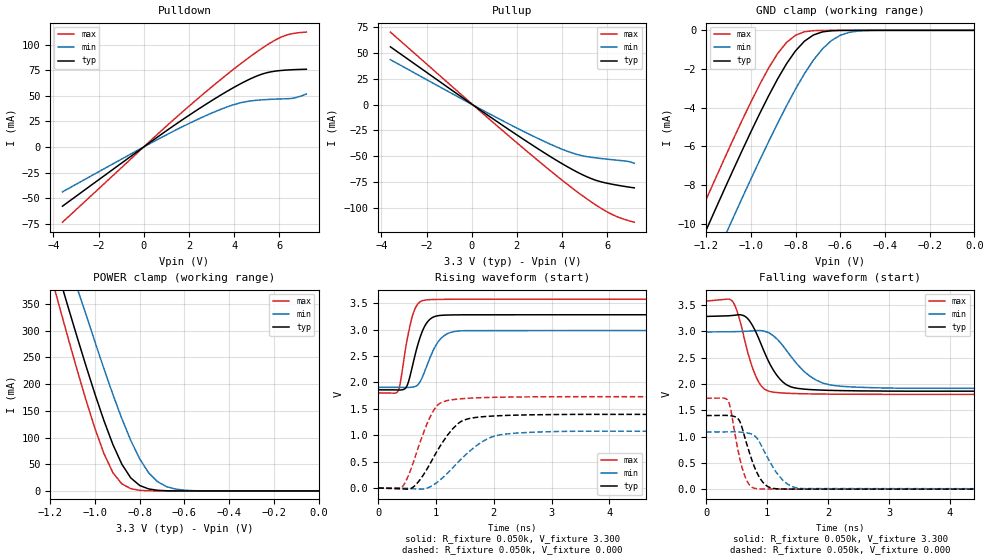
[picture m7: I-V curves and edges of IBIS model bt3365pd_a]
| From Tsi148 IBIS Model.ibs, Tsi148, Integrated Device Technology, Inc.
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|   MODEL bt3365pd_a
[Model]   bt3365pd_a
Model_type   I/O
Vinl  = 0.8V
Vinh  = 2.0V
Vref  = 0.0V
Rref  = 1k
Cref  = 10pF
Vmeas = 1.65V
| Values for delay from A to PAD (Tdo) are determined using
| Vref, Cref, Rref, and Vmeas.
|   INPUT TRANSITION ON DRIVER INPUT = 0.1ns
|   typ   min   max
| Tdo (rise)   1.63n   1.15n   2.34n
| Tdo (fall)   1.53n   1.15n   2.10n
|   INPUT TRANSITION ON DRIVER INPUT = 1.0ns
|   typ   min   max
| Tdo (rise)   1.84n   1.30n   2.60n
| Tdo (fall)   1.63n   1.25n   2.21n
|   typ   min   max
C_comp   1.29pF   1.27pF  1.30pF
[Temperature Range]   50.00   125.00   0.00
[Voltage Range]   3.300   3.000   3.600
|   typ   min   max
|[Supply]   VDD   1.80   1.65   1.95
|[Supply]   VDD330   3.30   3.00   3.60
[Add Submodel]
| Submodel Name   Mode
Up.bt3365pd_a   Non-Driving
Dn.bt3365pd_a   Non-Driving
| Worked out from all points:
|   slope of the pulldown table from 0 to 0.495 V, typ, clamps not added: 62.8 ohm
|   slope of the pullup table from 0 to 0.495 V, typ, clamps not added: 65.6 ohm
|   GND clamp passes 1 mA (typ) near -0.80 V on its own axis
|   POWER clamp passes 1 mA (typ) near -0.71 V on its own axis
|   rising waveform, R_fixture 0.050k, V_fixture 3.300: 20-80 % time 220ps typ, 268ps min, 176ps max; typ from 1.86 V to 3.29 V
|   falling waveform, R_fixture 0.050k, V_fixture 3.300: 20-80 % time 364ps typ, 510ps min, 262ps max; typ from 3.29 V to 1.86 V
|   rising waveform, R_fixture 0.050k, V_fixture 0.000: 20-80 % time 488ps typ, 655ps min, 355ps max; typ from 0 V to 1.4 V
|   falling waveform, R_fixture 0.050k, V_fixture 0.000: 20-80 % time 246ps typ, 336ps min, 182ps max; typ from 1.4 V to 0 V
[Pullup]   | Note: Vtable = Vcc - Vout
| Voltage   I(typ)   I(min)   I(max)
-3.6V     56.12mA    43.64mA    70.43mA
1.37V     -20.18mA   -15.67mA   -25.27mA
3.02V     -44.1mA    -33.79mA   -55.87mA
4.12V     -58.9mA    -44.36mA   -75.46mA
4.67V     -65.54mA   -48.47mA   -84.72mA
5.11V     -70.21mA   -50.58mA   -91.74mA
5.88V     -75.84mA   -52.74mA   -102.7mA
6.54V     -78.66mA   -54.24mA   -109.8mA
6.87V     -79.84mA   -55mA      -112.2mA
7.2V      -80.88mA   -56.98mA   -114.3mA
[Pulldown]   | Note: Vtable = Vout
| Voltage   I(typ)   I(min)   I(max)
-3.6V     -57.91mA   -43.93mA   -73.58mA
1.35V     21.13mA    15.75mA    27.16mA
2.89V     43.61mA    31.96mA    56.47mA
3.99V     58.18mA    41.33mA    76.18mA
4.54V     64.64mA    44.3mA     85.49mA
5.09V     70.03mA    45.79mA    94.25mA
5.53V     72.96mA    46.44mA    100.7mA
5.97V     74.5mA     46.85mA    106.2mA
6.3V      75.12mA    47.08mA    109.2mA
6.63V     75.52mA    47.72mA    111mA
7.2V      75.96mA    51.68mA    112.3mA
[POWER_Clamp]   | Note: Vtable = Vcc - Vout
| Voltage   I(typ)   I(min)   I(max)
-3.6V     3.946A     3.816A     4.188A
-1.2V     455.7mA    530.2mA    407.9mA
-1.16V    400.6mA    479.4mA    346.3mA
-1.12V    343.9mA    429.2mA    285.8mA
-1.08V    288.1mA    379.7mA    226.7mA
-1.04V    233.7mA    330.1mA    169.8mA
-1V       181.1mA    278.8mA    116.7mA
-920mV    86.97mA    180.7mA    34.22mA
-840mV    24.39mA    94.6mA     4.235mA
-720mV    1.176mA    17.25mA    44uA
-600mV    19uA       1.348mA    0A
0V        0A         0A         0A
[GND_Clamp]   | Note: Vtable = Vout
| Voltage   I(typ)   I(min)   I(max)
-3.6V     -76.49mA   -78.79mA   -75.06mA
-1.28V    -12.45mA   -14.94mA   -10.87mA
-1.24V    -11.4mA    -13.88mA   -9.809mA
-1.2V     -10.35mA   -12.84mA   -8.759mA
-1.12V    -8.273mA   -10.76mA   -6.689mA
-1.08V    -7.253mA   -9.729mA   -5.675mA
-920mV    -3.381mA   -5.752mA   -1.944mA
-840mV    -1.725mA   -3.901mA   -626uA
-760mV    -561uA     -2.244mA   -74uA
-640mV    -23uA      -536uA     -1uA
-520mV    0A         -38uA      0A
0V        0A         0A         0A
[Ramp]
| variable   typ   min   max
  dV/dt_r   0.84/0.49n   0.65/0.66n   1.04/0.36n
  dV/dt_f   0.86/0.36n   0.65/0.51n   1.07/0.26n
R_load = 0.050k
[Rising Waveform]
R_fixture = 0.050k
V_fixture = 3.300
V_fixture_min = 3.000
V_fixture_max = 3.600
|   time   V(typ)   V(min)   V(max)
0s        1.86V      1.907V     1.802V
340ps     1.857V     1.907V     1.831V
390ps     1.858V     1.906V     2.042V
480ps     1.902V     1.905V     2.687V
640ps     2.529V     1.924V     3.402V
750ps     2.931V     2.067V     3.542V
860ps     3.156V     2.366V     3.566V
1.11ns    3.272V     2.859V     3.573V
1.5ns     3.281V     2.981V     3.577V
19.9ns    3.286V     2.991V     3.579V
[Falling Waveform]
R_fixture = 0.050k
V_fixture = 3.300
V_fixture_min = 3.000
V_fixture_max = 3.600
|   time   V(typ)   V(min)   V(max)
0s        3.286V     2.991V     3.579V
430ps     3.304V     2.995V     3.575V
530ps     3.317V     2.998V     3.305V
660ps     3.268V     3.004V     2.708V
780ps     3.071V     3.012V     2.249V
900ps     2.763V     3.015V     1.972V
1.22ns    2.083V     2.784V     1.832V
1.8ns     1.889V     2.077V     1.811V
2.38ns    1.872V     1.945V     1.805V
19.9ns    1.86V      1.907V     1.802V
[Rising Waveform]
R_fixture = 0.050k
V_fixture = 0.000
V_fixture_min = 0.000
V_fixture_max = 0.000
|   time   V(typ)   V(min)   V(max)
0s        0V         0V         0V
400ps     -12mV      -1mV       2mV
610ps     23mV       -13mV      494mV
840ps     353mV      -4mV       1.205V
1ns       664mV      93mV       1.536V
1.2ns     1.004V     283mV      1.658V
1.44ns    1.265V     555mV      1.692V
2ns       1.365V     981mV      1.718V
2.96ns    1.391V     1.067V     1.729V
19.9ns    1.4V       1.089V     1.731V
[Falling Waveform]
R_fixture = 0.050k
V_fixture = 0.000
V_fixture_min = 0.000
V_fixture_max = 0.000
|   time   V(typ)   V(min)   V(max)
0s        1.4V       1.089V     1.731V
360ps     1.402V     1.091V     1.683V
530ps     1.331V     1.087V     704mV
620ps     1.047V     1.079V     299mV
720ps     660mV      1.058V     70mV
850ps     277mV      946mV      6mV
1.01ns    51mV       597mV      2mV
1.25ns    3mV        180mV      1mV
1.57ns    2mV        11mV       1mV
19.9ns    0V         0V         0V
